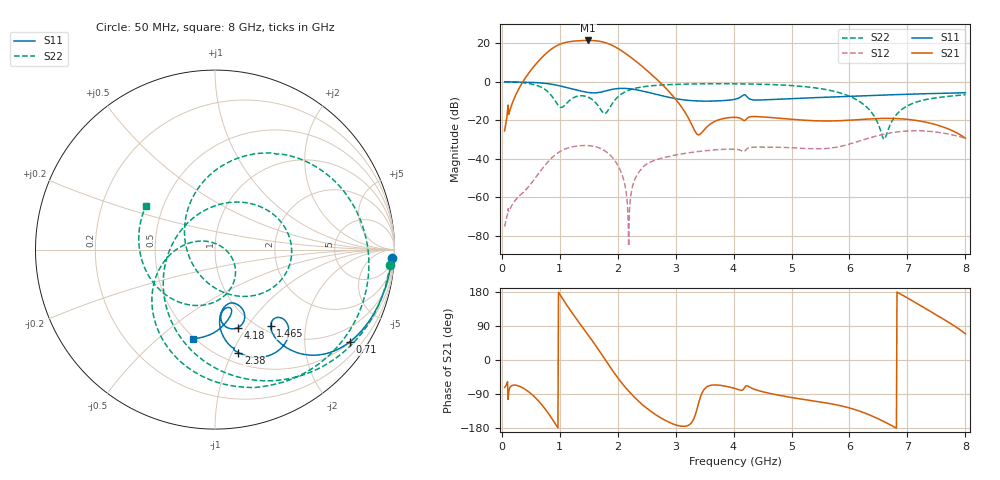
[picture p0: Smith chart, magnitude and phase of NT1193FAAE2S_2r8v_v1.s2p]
! Created Wed Jun 21 19:34:22 2023
# hz S ma R 50
! 2 Port Network Data from SP9.SP block
! freq  magS11  angS11  magS21  angS21  magS12  angS12  magS22  angS22
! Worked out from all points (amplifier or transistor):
!   856 points, 50 MHz to 8 GHz, reference 50 ohm
!   highest |S21| = 21.3 dB at 1.49 GHz (marker M1)
!   |S21| within 3 dB of that: 933.7 MHz to 1.936 GHz (1.002 GHz wide, 69.9 % of centre)
!   unconditionally stable (mu >= 1): start of sweep to end of sweep
!   at 1.285 GHz: K = 1.46, MAG = 23.2 dB, |S12| = -33.5 dB
!   at 3.73 GHz: K = 61.11, MAG = -13.2 dB, |S12| = -35.3 dB
!   at 8 GHz: K = 255.70, MAG = -27.1 dB, |S12| = -29.4 dB
!   lowest NFmin = 0.40 dB at 590 MHz
!   S11 on the Smith chart (normalised r, x): 50 MHz: 13, -41; 710 MHz: 0.53, -3.15; 1.465 GHz: 1.10, -1.30; 2.38 GHz: 0.60, -1.06; 4.18 GHz: 0.84, -0.92; 8 GHz: 0.49, -0.66
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5e7  0.9859 -2.6  0.0525 -72.4  0.0001721 99.0  0.9815 -5.0
4.9e8  0.9515 -23.1  1.845 -87.0  0.002097 126.6  0.8742 -50.0
7.1e8  0.9097 -34.4  4.451 -121.5  0.005738 130.4  0.6756 -87.3
8.8e8  0.8416 -43.7  7.329 -157.8  0.01104 113.8  0.3907 -136.1
1.06e9  0.7331 -51.5  9.889 159.4  0.01691 87.0  0.2224 109.0
1.225e9  0.6357 -55.0  11.05 122.1  0.02036 62.0  0.3715 34.4
1.375e9  0.5626 -55.4  11.48 90.5  0.02175 40.6  0.4275 -3.6
1.465e9  0.5283 -54.0  11.59 71.8  0.02185 27.8  0.4064 -24.1
1.49e9  0.5209 -53.3  11.6 66.5  0.02176 24.2  0.3935 -30.0
1.61e9  0.5074 -49.0  11.42 40.6  0.02051 6.1  0.2938 -62.2
1.71e9  0.5313 -45.8  10.89 18.0  0.01823 -9.8  0.1856 -104.5
1.82e9  0.5846 -46.0  9.801 -7.2  0.01443 -27.6  0.1656 170.3
1.95e9  0.6433 -51.5  8.007 -36.0  0.008987 -47.5  0.3269 110.9
2.17e9  0.6568 -65.5  4.916 -78.6  0.0005948 -78.6  0.5759 67.7
2.38e9  0.5884 -77.2  2.804 -111.2  0.004741 89.7  0.7071 43.9
2.7e9  0.4518 -85.8  1.051 -148.7  0.009722 79.2  0.801 20.4
3.38e9  0.3128 -77.4  0.04215 -123.6  0.01522 59.0  0.8685 -11.3
4.03e9  0.348 -66.1  0.1176 -75.4  0.01758 37.2  0.8725 -36.0
4.18e9  0.4533 -73.6  0.09723 -75.3  0.01522 39.9  0.8679 -41.7
5.35e9  0.3787 -77.0  0.09681 -107.4  0.01812 -36.5  0.7025 -97.2
6.68e9  0.4503 -88.2  0.1107 -169.2  0.04576 150.5  0.0634 -4.4
8e9  0.5109 -103.7  0.0338 68.9  0.03388 23.0  0.4548 147.8
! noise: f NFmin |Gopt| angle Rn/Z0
5e+07  2.392  0.9627  2.963  14.27
1e+09  0.4608  0.692  35.03  0.2472
1.525e+09  0.6503  0.6308  50.09  0.2429
2.3e+09  1.228  0.5327  70.09  0.2718
3.25e+09  14.59  0.3235  80.57  9.474
4.2e+09  13.75  0.4563  79.91  10.01
5.15e+09  16.03  0.3663  77.19  14.83
6.1e+09  18.62  0.4153  83.09  27.89
7.05e+09  18.64  0.4654  91.64  27.75
8e+09  27.17  0.5117  103.5  181
